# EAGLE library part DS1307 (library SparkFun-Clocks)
Maxim DS1307 - I2C Real-time clock (RTC) The DS1307 serial real-time clock (RTC) is a low-power, full binary-coded decimal (BCD) clock/calendar plus 56 bytes of NV SRAM. Address and data are transferred serially through an I2C, bidirectional bus. The clock/calendar provides seconds, minutes, hours, day, date, month, and year information. SparkFun Products: Real Time Clock Module (BOB-12708) Datasheet
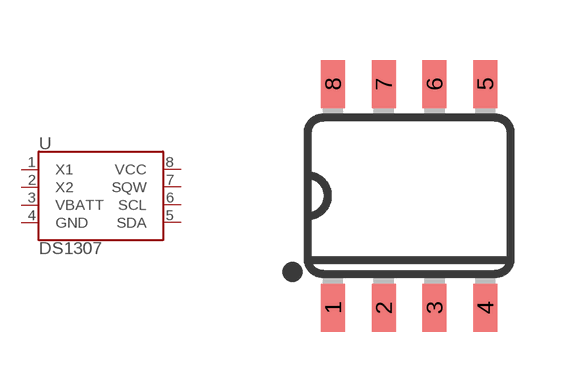
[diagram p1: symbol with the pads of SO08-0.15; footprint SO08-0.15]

Designator prefix U

## DS1307Z (PROD_ID: IC-08138)  [SO08-0.15]
1  X1
2  X2
3  VBATT
4  GND
5  SDA
6  SCL
7  SQW
8  VCC

## Footprint SO08-0.15 (pad centres in mm)
8-Pin SOIC 150mil 0.154" (3.9mm) width. Fits JEDEC packages (narrow SOIC-8). Used by DS1077 and DS1307 programmable oscillators
smd 0.6 x 1.2: 1 -1.905,-2.8; 2 -0.635,-2.8; 3 0.635,-2.8; 4 1.905,-2.8; 5 1.905,2.8; 6 0.635,2.8; 7 -0.635,2.8; 8 -1.905,2.8

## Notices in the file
Licensing: Creative Commons ShareAlike 4.0 International - https://creativecommons.org/licenses/by-sa/4.0
